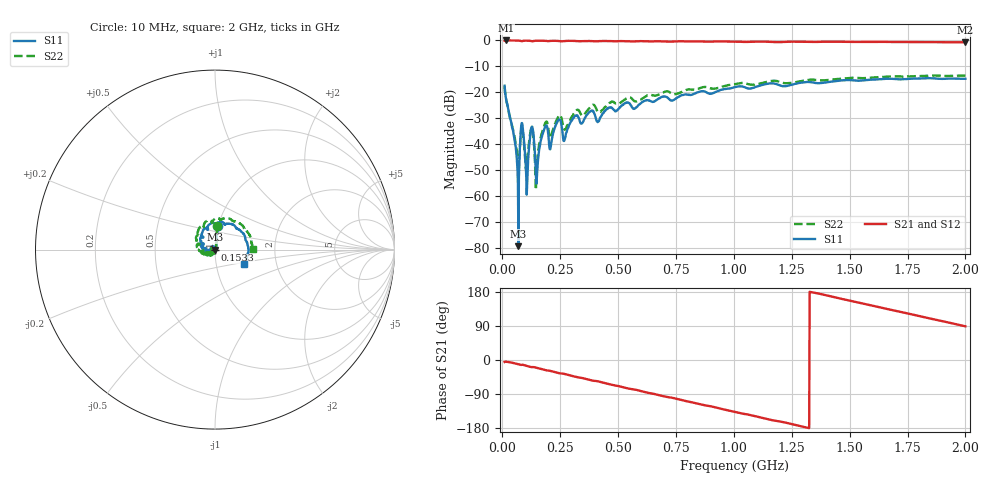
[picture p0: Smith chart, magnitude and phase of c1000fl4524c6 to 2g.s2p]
!Agilent Technologies,N5234A,MY52241123,A.10.00.00
!Agilent N5234A: A.10.00.00
!Date: Tuesday, April 16, 2019 15:10:19
!Correction: S11(Full 2 Port(1,2))
!S21(Full 2 Port(1,2))
!S12(Full 2 Port(1,2))
!S22(Full 2 Port(1,2))
!S2P File: Measurements: S11, S21, S12, S22:
# Hz S  dB  R 50
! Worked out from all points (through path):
!   1001 points, 10 MHz to 2 GHz, reference 50 ohm
!   highest |S21| = -0.04 dB at 15.97 MHz (marker M1); lowest = -0.8 dB at 2 GHz (marker M2)
!   group delay of S21, straight-line fit = 374 ps
!   lowest |S11| = -79.2 dB at 69.7 MHz (marker M3), VSWR 1.00, Z = 50 - j0.0109 ohm
!   |S11| at or under -10 dB: start of sweep to end of sweep
!   |S22| runs from -57.5 to -13.5 dB; largest |S21 - S12| = 0.0053
!   S11 on the Smith chart (normalised r, x): 10 MHz: 1.00, +0.27; 153.3 MHz: 1.00, -0.01; 2 GHz: 1.37, -0.23
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1e7  -17.46 82.6  -0.13 -5.2  -0.09 -5.4  -17.61 85.0
1.597e7  -22.49 83.0  -0.04 -4.6  -0.03 -4.6  -22.20 84.4
5.179e7  -37.63 67.9  -0.06 -8.5  -0.06 -8.5  -36.64 64.3
6.174e7  -44.23 62.7  -0.07 -10.0  -0.07 -10.0  -41.88 46.9
6.97e7  -79.18 -98.8  -0.09 -11.2  -0.09 -11.2  -50.63 -26.8
8.562e7  -31.85 140.1  -0.31 -12.5  -0.31 -12.5  -32.89 148.4
1.0353e8  -52.60 36.2  -0.11 -15.1  -0.11 -15.2  -49.92 -9.2
1.2741e8  -33.22 174.5  -0.33 -18.6  -0.33 -18.6  -33.24 -165.5
1.4333e8  -47.35 73.8  -0.16 -19.9  -0.16 -19.9  -53.46 77.8
1.5328e8  -47.02 -77.0  -0.13 -21.5  -0.13 -21.5  -43.76 -68.7
1.8512e8  -33.28 -131.6  -0.20 -26.7  -0.20 -26.7  -31.88 -112.7
2.09e8  -41.09 -128.1  -0.20 -29.0  -0.20 -29.0  -37.40 -123.4
2.4283e8  -30.69 -141.7  -0.25 -34.5  -0.25 -34.5  -29.23 -124.9
2.687e8  -38.36 -139.5  -0.25 -36.8  -0.25 -36.8  -34.39 -140.4
3.1248e8  -29.22 -138.7  -0.22 -43.8  -0.22 -43.8  -27.73 -124.3
3.4233e8  -32.06 -150.7  -0.30 -47.1  -0.29 -47.1  -28.84 -146.0
3.8412e8  -27.03 -158.3  -0.31 -53.6  -0.31 -53.6  -25.34 -143.7
6.7466e8  -22.43 170.6  -0.35 -92.4  -0.35 -92.4  -20.89 176.0
1.005e9  -18.00 122.1  -0.49 -137.2  -0.48 -137.2  -16.85 129.2
1.33733e9  -16.15 71.1  -0.61 178.7  -0.61 178.7  -15.12 85.1
1.66966e9  -14.78 25.9  -0.61 133.6  -0.61 133.6  -13.92 45.4
2e9  -14.77 -26.9  -0.75 88.9  -0.75 88.9  -13.60 1.6
